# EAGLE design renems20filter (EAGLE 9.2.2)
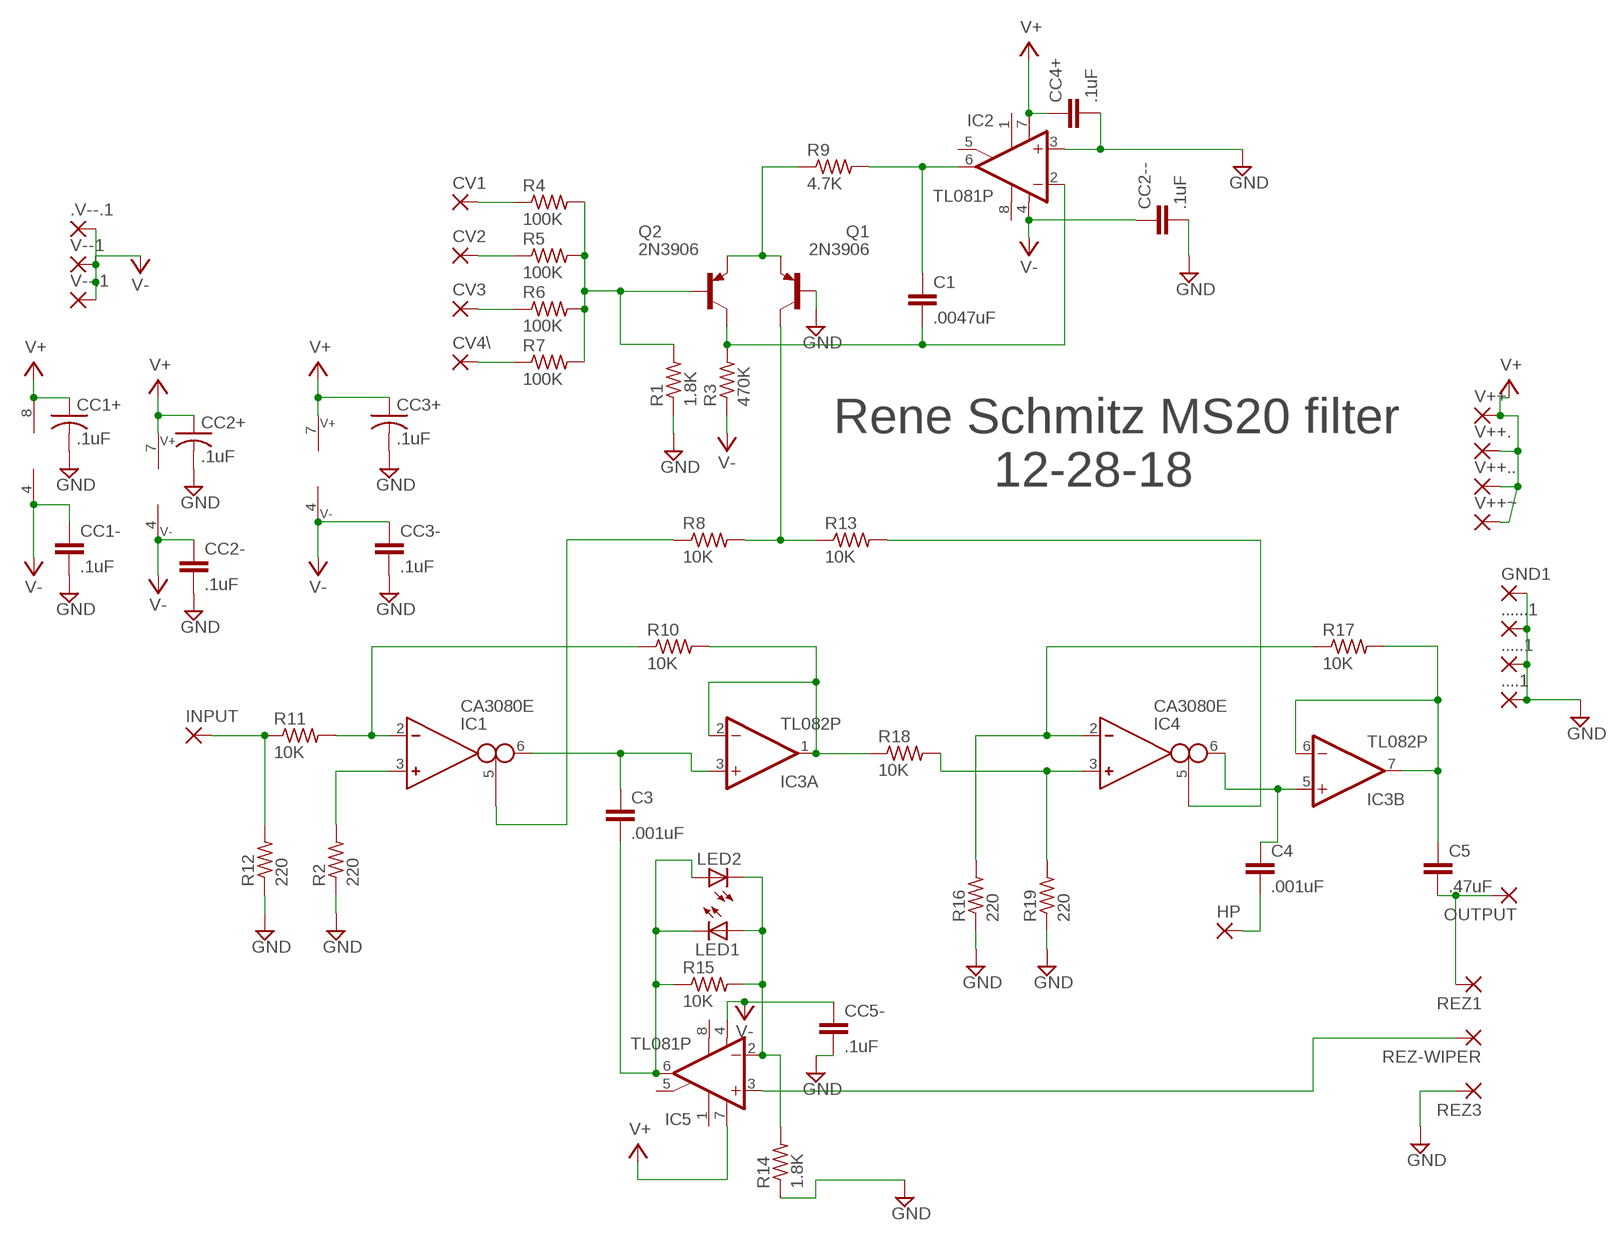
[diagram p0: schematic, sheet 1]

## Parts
....1  3,17/1,3  [3,17/1,3]
.....1  3,17/1,3  [3,17/1,3]
......1  3,17/1,3  [3,17/1,3]
.V--.1  3,17/1,3  [3,17/1,3]
C1  .0047uF  C5/2.5  [C5B2.5]
C3  .001uF  C5/2.5  [C5B2.5]
C4  .001uF  C5/2.5  [C5B2.5]
C5  .47uF  C5/2.5  [C5B2.5]
CC1+  .1uF  C-US050-025X075  [C050-025X075]
CC1-  .1uF  C2.5/2  [C2.5-2]
CC2+  .1uF  C-US025-024X044  [C025-024X044]
CC2-  .1uF  C2.5/2  [C2.5-2]
CC2--  .1uF  C2.5/2  [C2.5-2]
CC3+  .1uF  C-US050-025X075  [C050-025X075]
CC3-  .1uF  C2.5/2  [C2.5-2]
CC4+  .1uF  C2.5/2  [C2.5-2]
CC5-  .1uF  C2.5/2  [C2.5-2]
CV1  3,17/1,3  [3,17/1,3]
CV2  3,17/1,3  [3,17/1,3]
CV3  3,17/1,3  [3,17/1,3]
CV4\  3,17/1,3  [3,17/1,3]
GND1  3,17/1,3  [3,17/1,3]
HP  3,17/1,3  [3,17/1,3]
IC1  CA3080E  [DIL08]
IC2  TL081P  [DIL08]
IC3  TL082P  [DIL08]
IC4  CA3080E  [DIL08]
IC5  TL081P  [DIL08]
INPUT  3,17/1,3  [3,17/1,3]
LED1  LED3MM  [LED3MM]
LED2  LED3MM  [LED3MM]
OUTPUT  3,17/1,3  [3,17/1,3]
Q1  2N3906  [TO92]
Q2  2N3906  [TO92]
R1  1.8K  R-US_0204/7  [0204/7]
R2  220  R-US_0204/7  [0204/7]
R3  470K  R-US_0204/7  [0204/7]
R4  100K  R-US_0204/7  [0204/7]
R5  100K  R-US_0204/7  [0204/7]
R6  100K  R-US_0204/7  [0204/7]
R7  100K  R-US_0204/7  [0204/7]
R8  10K  R-US_0204/7  [0204/7]
R9  4.7K  R-US_0204/7  [0204/7]
R10  10K  R-US_0204/7  [0204/7]
R11  10K  R-US_0204/7  [0204/7]
R12  220  R-US_0204/7  [0204/7]
R13  10K  R-US_0207/12  [0207/12]
R14  1.8K  R-US_0204/7  [0204/7]
R15  10K  R-US_0204/7  [0204/7]
R16  220  R-US_0204/7  [0204/7]
R17  10K  R-US_0204/7  [0204/7]
R18  10K  R-US_0204/7  [0204/7]
R19  220  R-US_0204/7  [0204/7]
REZ1  3,17/1,3  [3,17/1,3]
REZ3  3,17/1,3  [3,17/1,3]
REZ-WIPER  3,17/1,3  [3,17/1,3]
V++  3,17/1,3  [3,17/1,3]
V++.  3,17/1,3  [3,17/1,3]
V++..  3,17/1,3  [3,17/1,3]
V++~  3,17/1,3  [3,17/1,3]
V--1  3,17/1,3  [3,17/1,3]
V--.1  3,17/1,3  [3,17/1,3]

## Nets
GND: ....1.1(P) .....1.1(P) ......1.1(P) CC1+.2 CC1-.2 CC2+.2 CC2--.2 CC2-.2 CC3+.2 CC3-.2 CC4+.2 CC5-.2 GND1.1(P) IC2.3(+IN) Q1.2(B) R1.1 R2.1 R12.1 R14.1 R16.1 R19.1 REZ3.1(P)
N$1: Q2.2(B) R1.2 R4.2 R5.2 R6.2 R7.2
N$2: Q1.3(E) Q2.3(E) R9.1
N$3: C1.1 IC2.6(OUT) R9.2
N$4: C1.2 IC2.2(-IN) Q2.1(C) R3.2
N$5: Q1.1(C) R8.2 R13.1
N$6: INPUT.1(P) R11.1 R12.2
N$7: IC1.2(IN_N) R10.1 R11.2
N$8: IC1.3(IN_P) R2.2
N$9: IC1.5(I_BIAS) R8.1
N$10: IC4.2(IN_N) R16.2 R17.1
N$11: C5.1 IC3.6(B:-IN) IC3.7(B:OUT) R17.2
N$12: C3.1 IC1.6(OUT) IC3.3(A:+IN)
N$13: C3.2 IC5.6(OUT) LED1.K(C) LED2.A R15.1
N$14: IC5.2(-IN) LED1.A LED2.K(C) R14.2 R15.2
N$15: IC4.5(I_BIAS) R13.2
N$16: C4.1 IC3.5(B:+IN) IC4.6(OUT)
N$17: IC3.1(A:OUT) IC3.2(A:-IN) R10.2 R18.1
N$18: C4.2 HP.1(P)
N$19: IC4.3(IN_P) R18.2 R19.2
N$20: C5.2 OUTPUT.1(P) REZ1.1(P)
N$21: CV1.1(P) R4.1
N$22: IC5.3(+IN) REZ-WIPER.1(P)
N$23: CV2.1(P) R5.1
N$24: CV3.1(P) R6.1
N$25: CV4\.1(P) R7.1
V+: CC1+.1 CC2+.1 CC3+.1 CC4+.1 IC1.7(V+) IC2.7(V+) IC3.8(P:V+) IC4.7(V+) IC5.7(V+) V++.1(P) V++..1(P) V++...1(P) V++~.1(P)
V-: .V--.1.1(P) CC1-.1 CC2--.1 CC2-.1 CC3-.1 CC5-.1 IC1.4(V-) IC2.4(V-) IC3.4(P:V-) IC4.4(V-) IC5.4(V-) R3.1 V--1.1(P) V--.1.1(P)
Unconnected: IC2.1(ON1) IC2.5(ON2) IC2.8(OPT) IC5.1(ON1) IC5.5(ON2) IC5.8(OPT)

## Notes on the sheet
- Rene Schmitz MS20 filter
- 12-28-18

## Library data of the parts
....1 .....1 ......1 .V--.1 GND1 V++ V++. V++.. V++~ V--1 V--.1 = wirepad-NONAMES:3,17/1,3: THROUGH-HOLE PAD
C1 C3-C5 CC1- CC2- CC2-- CC3- CC4+ CC5- = capacitor-wima:C: CAPACITOR
CC1+ CC2+ CC3+ = rcl:C-US: CAPACITOR, American symbol; SPICEPREFIX: C
CV1-CV3 CV4\ HP INPUT OUTPUT REZ1 REZ3 REZ-WIPER = wirepad:3,17/1,3: THROUGH-HOLE PAD
IC1 IC4 = ota:CA3080: OTA
IC2 IC5 = linear:TL081: OP AMP
IC3 = linear:TL082: OP AMP Data sheet; DATA_SHEET: <a href="http://www.ti.com/lit/ds/symlink/tl084a.pdf"> Data sheet </a>
LED1 LED2 = led:LED: LED
Q1 Q2 = transistor-pnp:2N3906: PNP Transistor
R1-R12 R14-R19 = rcl:R-US_: RESISTOR, American symbol
R13 = resistor:R-US_: RESISTOR, American symbol

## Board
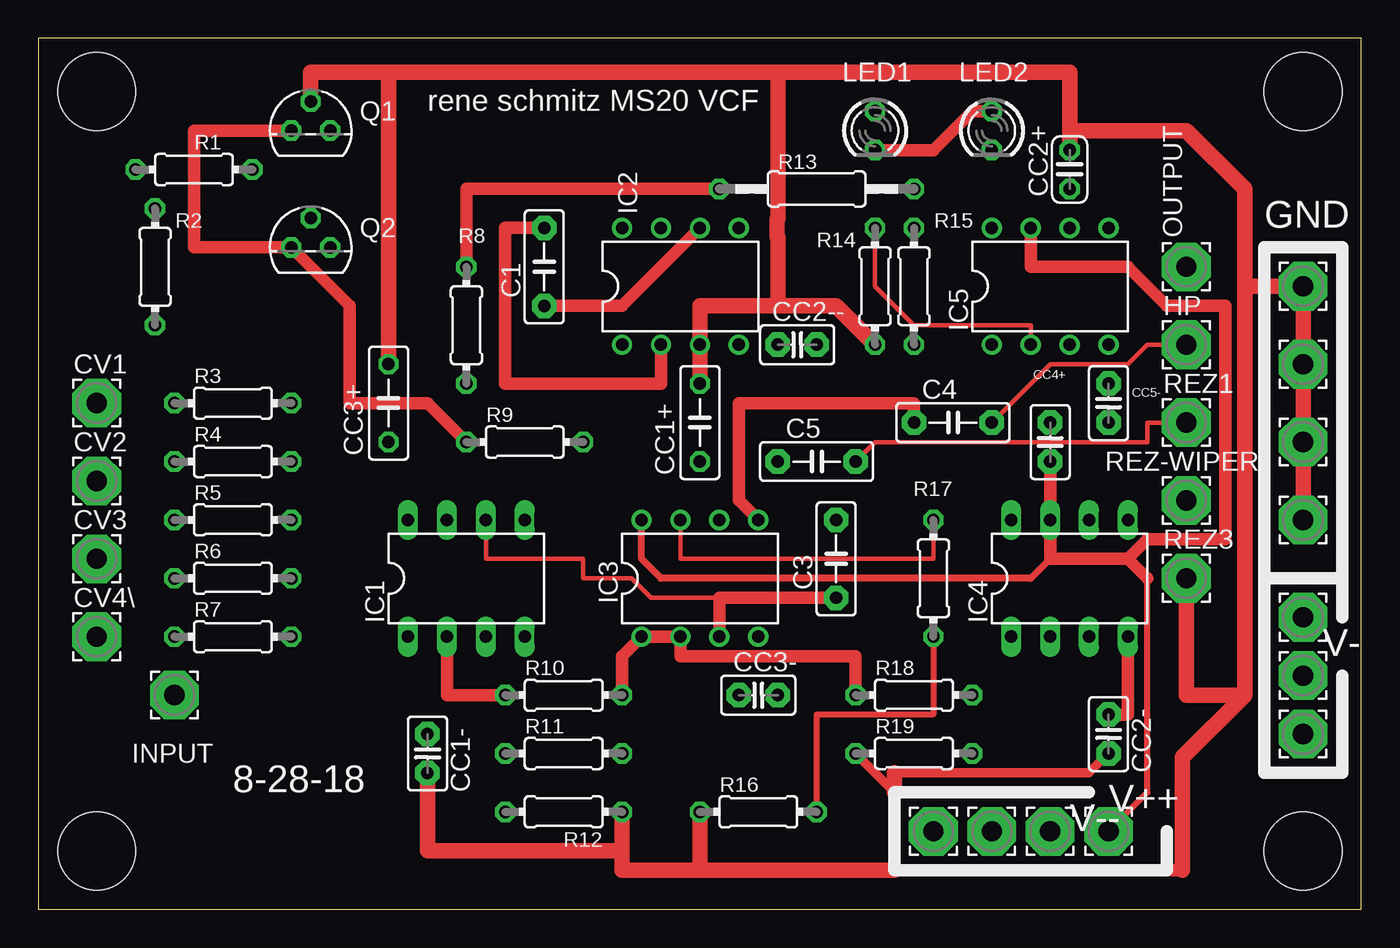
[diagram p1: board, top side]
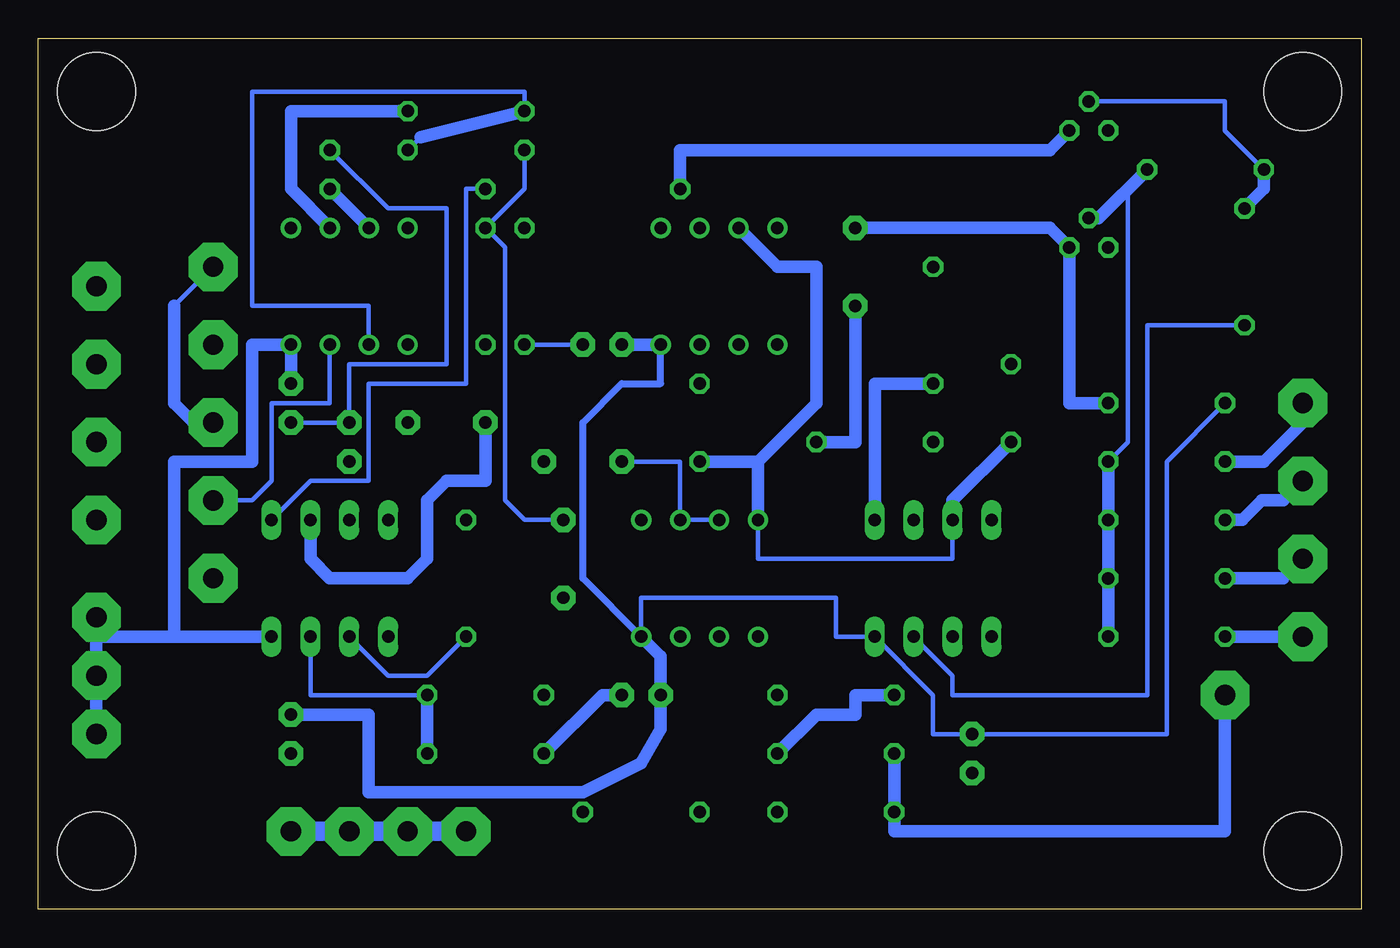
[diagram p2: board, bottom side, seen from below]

Size 86.34 x 56.82 mm. Coordinates in mm from the lower left corner, seen from the top.
Outline: 0,0 86.34,0 86.34,56.82 0,56.82 0,0
Copper layers (1*16): Top 0.035mm / dielectric 1.5mm / Bottom 0.035mm
Design rules "default": minimum track width 6mil, minimum drill 0.35mm, track to track 6mil, track to pad 6mil, pad to pad 6mil, via to via 6mil, smd to smd 6mil, copper to edge 40mil, drill to drill 6mil, minimum pad ring 10mil, minimum via ring 8mil, stop-mask expansion 4mil, vias tented up to drill 0mil, thermal gap 10mil
Holes 5.08 mm at 3.81,53.34 3.81,3.81 82.55,3.81 82.55,53.34

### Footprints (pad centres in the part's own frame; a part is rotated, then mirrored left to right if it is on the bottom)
3,17/1,3 = drill 1.321 pad 3.175 octagon: 1 0,0
C5B2.5 = drill 0.813 pad 1.6 octagon: 1 -2.54,0; 2 2.54,0
C050-025X075 = drill 0.813 octagon: 1 -2.54,0; 2 2.54,0
C2.5-2 = drill 0.813 pad 1.6 octagon: 1 -1.27,0; 2 1.27,0
C025-024X044 = drill 0.813 octagon: 1 -1.27,0; 2 1.27,0
DIL08 = drill 0.813 long: 1 -3.81,-3.81; 2 -1.27,-3.81; 3 1.27,-3.81; 4 3.81,-3.81; 5 3.81,3.81; 6 1.27,3.81; 7 -1.27,3.81; 8 -3.81,3.81
DIL08' = drill 0.813 pad 1.27: 1 -3.81,-3.81; 2 -1.27,-3.81; 3 1.27,-3.81; 4 3.81,-3.81; 5 3.81,3.81; 6 1.27,3.81; 7 -1.27,3.81; 8 -3.81,3.81
LED3MM = drill 0.813 octagon: A -1.27,0; K 1.27,0
TO92 = drill 0.813 octagon: 1 1.27,0; 2 0,1.905; 3 -1.27,0
0204/7 = drill 0.813 octagon: 1 -3.81,0; 2 3.81,0
0207/12 = drill 0.813 octagon: 1 -6.35,0; 2 6.35,0

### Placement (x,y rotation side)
....1  82.55,25.4 0 top
.....1  82.55,30.48 0 top
......1  82.55,35.56 0 top
.V--.1  82.55,11.43 0 top
C1  33.02,41.91 90 top
C3  52.07,22.86 90 top
C4  59.69,31.75 0 top
C5  50.8,29.21 0 top
CC1+  43.18,31.75 90 top
CC1-  25.4,10.16 270 top
CC2+  67.31,48.26 90 top
CC2-  69.85,11.43 270 top
CC2--  49.53,36.83 0 top
CC3+  22.86,33.02 90 top
CC3-  46.99,13.97 0 top
CC4+  66.04,30.48 90 top
CC5-  69.85,33.02 270 top
CV1  3.81,33.02 0 top
CV2  3.81,27.94 0 top
CV3  3.81,22.86 0 top
CV4\  3.81,17.78 0 top
GND1  82.55,40.64 0 top
HP  74.93,36.83 0 top
IC1  27.94,21.59 0 top
IC2  TL081P  [DIL08']  41.91,40.64 0 top
IC3  TL082P  [DIL08']  43.18,21.59 0 top
IC4  67.31,21.59 0 top
IC5  TL081P  [DIL08']  66.04,40.64 0 top
INPUT  8.89,13.97 0 top
LED1  54.61,50.8 270 top
LED2  62.23,50.8 270 top
OUTPUT  74.93,41.91 0 top
Q1  17.78,50.8 0 top
Q2  17.78,43.18 0 top
R1  10.16,48.26 0 top
R2  7.62,41.91 270 top
R3  12.7,33.02 0 top
R4  12.7,29.21 0 top
R5  12.7,25.4 0 top
R6  12.7,21.59 0 top
R7  12.7,17.78 0 top
R8  27.94,38.1 90 top
R9  31.75,30.48 0 top
R10  34.29,13.97 0 top
R11  34.29,10.16 0 top
R12  34.29,6.35 180 top
R13  50.8,46.99 0 top
R14  54.61,40.64 90 top
R15  57.15,40.64 270 top
R16  46.99,6.35 0 top
R17  58.42,21.59 90 top
R18  57.15,13.97 0 top
R19  57.15,10.16 0 top
REZ1  74.93,31.75 0 top
REZ3  74.93,21.59 0 top
REZ-WIPER  74.93,26.67 0 top
V++  58.42,5.08 0 top
V++.  69.85,5.08 0 top
V++..  62.23,5.08 0 top
V++~  66.04,5.08 0 top
V--1  82.55,15.24 0 top
V--.1  82.55,19.05 0 top

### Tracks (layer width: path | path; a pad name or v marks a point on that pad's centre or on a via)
GND
  Top 0.61: 55.88,7.62 R19.1 | CC2-.2 68.58,8.89 64.77,8.89 55.88,8.89
  Top 0.813: 55.88,2.54 55.88,7.62 | 54.61,2.54 74.68,2.54
  Top 1.016: 55.88,2.54 54.61,2.54 50.8,2.54 43.18,2.54 | 43.18,2.54 R16.1 | 78.74,40.64 78.74,13.97 | 78.74,40.64 78.74,46.99 74.93,50.8 67.31,50.8 CC2+.2 67.31,54.61 48.26,54.61 | 38.1,3.81 R12.1 | 48.26,54.61 22.86,54.61 | 22.86,54.61 17.78,54.61 Q1.2 | 48.26,39.37 43.18,39.37 IC2.3 CC1+.2 | 48.26,39.37 52.07,39.37 R14.1 | 38.1,3.81 25.4,3.81 CC1-.2 | 48.26,39.37 48.26,43.85 48.21,43.9 48.21,45 48.26,45.05 48.26,54.61 | CC3+.2 22.86,54.61 | 78.74,40.64 GND1.1 ......1.1 .....1.1 ....1.1 | 55.88,7.62 55.88,8.89 | 38.1,3.81 38.1,2.54 43.18,2.54 | 78.74,13.97 74.93,13.97 REZ3.1 | 74.68,2.54 74.68,9.91 78.74,13.97
  Bottom 0.305: Q1.2 8.89,52.7 8.89,50.8 R1.1 | CC2+.2 63.5,45.72 59.69,45.72 59.69,35.56 66.04,35.56 CC4+.2 CC5-.2 | CC2--.2 R14.1
  Bottom 0.813: R1.1 6.35,46.99 R2.1 | R19.1 49.53,13.97 CC3-.2
N$1
  Bottom 0.305: Q2.2 17.15,45.09 | R4.2 15.24,30.48 15.24,46.99 R1.2
  Bottom 0.813: R4.2 R5.2 R6.2 R7.2 | 17.15,45.09 R1.2
N$2
  Top 0.813: Q1.3 10.16,50.8 10.16,43.18 Q2.3 20.32,39.37 20.32,33.02 25.4,33.02 R9.1
N$3
  Top 0.813: C1.1 38.1,39.37 IC2.6
  Bottom 0.813: C1.1 33.02,30.48 R9.2
N$4
  Top 0.813: IC2.2 40.64,34.29 30.48,34.29 30.48,44.45 C1.2
  Bottom 0.813: C1.2 20.32,44.45 Q2.1 19.05,33.02 R3.2
N$5
  Top 0.813: R8.2 27.94,46.99 R13.1
  Bottom 0.813: R13.1 44.45,49.53 20.32,49.53 Q1.1
N$6
  Bottom 0.813: R11.1 R12.2 30.48,5.08 8.89,5.08 INPUT.1
N$7
  Top 0.813: R10.1 26.67,13.97 IC1.2
  Bottom 0.813: R11.2 35.56,12.7 33.02,12.7 33.02,13.97 R10.1
N$8
  Bottom 0.305: R2.2 13.97,38.1 13.97,13.97 26.67,13.97 26.67,15.24 IC1.3
N$9
  Bottom 0.813: IC1.5 31.75,34.29 R8.1
N$10
  Top 0.406: R17.1 58.42,12.7 50.8,12.7 R16.2
  Bottom 0.305: IC4.2 63.5,15.24 60.96,15.24 R17.1
N$11
  Top 0.305: R17.2 58.42,22.86 41.91,22.86 IC3.7
  Bottom 0.305: IC3.7 IC3.6 44.45,29.21 C5.1
N$12
  Top 0.305: 44.45,20.32 39.99,20.32 38.72,21.59 35.56,21.59 35.56,22.86 29.21,22.86 IC1.6
  Top 0.813: IC3.3 44.45,20.32 C3.1
N$13
  Top 0.813: LED1.K 58.42,49.53 60.96,52.07 LED2.A
  Bottom 0.305: C3.2 54.61,25.4 55.88,26.67 55.88,43.18 R15.1 54.61,46.99 LED1.K
  Bottom 0.813: IC5.6 69.85,46.99 69.85,52.07 LED2.A
N$14
  Top 0.305: IC5.2 64.77,38.1 57.15,38.1 | 57.15,38.1 R15.2 | 57.15,38.1 54.61,40.64 R14.2
  Bottom 0.305: IC5.2 64.77,39.37 72.39,39.37 72.39,53.34 54.61,53.34 LED1.A | LED2.K 61.38,50.38
  Bottom 0.813: 61.38,50.38 LED1.A
N$15
  Bottom 0.305: IC4.5 68.58,27.94 64.77,27.94 64.77,34.29 58.42,34.29 58.42,46.99 R13.2
N$16
  Top 0.813: IC3.5 45.72,26.67 45.72,33.02 57.15,33.02 C4.1
  Bottom 0.813: IC4.6 68.58,22.86 67.31,21.59 62.23,21.59 60.96,22.86 60.96,26.67 59.69,27.94 57.15,27.94 C4.1
N$17
  Top 0.813: R18.1 53.34,16.51 41.91,16.51 IC3.2 IC3.1 38.1,16.51 R10.2
N$18
  Top 0.305: HP.1 72.39,36.83 71.12,35.56 66.04,35.56 C4.2
N$19
  Bottom 0.305: R18.2 68.58,13.97 IC4.3
  Bottom 0.813: R19.2 R18.2
N$20
  Top 0.305: REZ1.1 72.39,31.75 72.39,30.48 54.61,30.48 C5.2
  Bottom 0.305: 77.47,39.37 OUTPUT.1 | REZ1.1 76.2,31.75
  Bottom 0.813: 76.2,31.75 77.47,33.02 77.47,39.37
N$21
  Bottom 0.305: CV1.1 3.17,32.38
  Bottom 0.813: R4.1 6.35,29.21 3.17,32.38
N$22
  Bottom 0.305: REZ-WIPER.1 72.39,26.67 71.12,27.94 71.12,33.02 67.31,33.02 IC5.3
N$23
  Bottom 0.813: R5.1 7.76,25.4 6.49,26.67 5.08,26.67 CV2.1
N$24
  Bottom 0.305: 5.08,21.59 CV3.1
  Bottom 0.813: R6.1 5.08,21.59
N$25
  Bottom 0.813: R7.1 CV4\.1
V+
  Top 0.406: V++..1 72.39,7.62 72.39,21.59
  Top 0.457: 66.04,22.86 64.77,21.59 40.64,21.59 39.37,22.86 IC3.8
  Top 0.813: 71.12,22.86 66.04,22.86 IC4.7 CC4+.1 | 71.12,22.86 72.39,24.13 77.47,24.13 77.47,39.37 73.66,39.37 71.12,41.91 64.77,41.91 IC5.7 | 72.39,21.59 71.12,22.86
  Bottom 0.305: IC3.8 39.37,22.86 26.67,22.86 IC1.7
  Bottom 0.813: IC5.7 CC2+.1 | CC3+.1 26.67,26.67 IC1.7 | IC3.8 39.37,29.21 | 39.37,29.21 CC1+.1 | IC2.7 38.1,41.91 35.56,41.91 35.56,33.02 39.37,29.21
  Bottom 1.27: V++..1 V++~.1 V++...1 V++.1
V-
  Top 0.813: CC2-.1 71.12,12.7 IC4.4
  Bottom 0.305: IC3.4 46.99,20.32 34.29,20.32 34.29,17.78 IC1.4 27.94,13.97 27.94,11.43 CC1-.1 12.7,11.43 12.7,29.21 R3.1
  Bottom 0.457: IC3.4 50.8,21.59 50.8,31.75 48.26,34.29 45.72,34.29 IC2.4
  Bottom 0.813: IC4.4 77.47,17.78 | IC3.4 45.72,16.51 CC3-.1 45.72,11.75 46.99,9.52 50.8,7.62 64.77,7.62 64.77,12.7 CC2-.1 | 77.47,17.78 77.47,29.21 72.39,29.21 72.39,36.83 IC5.4 CC5-.1 | V--.1.1 82.55,17.78 | 82.55,17.78 V--1.1 .V--.1.1 | 77.47,17.78 82.55,17.78 | CC2--.1 IC2.4

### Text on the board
tNames: rene schmitz MS20 VCF | GND | V- | 8-28-18 | V++ | V--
